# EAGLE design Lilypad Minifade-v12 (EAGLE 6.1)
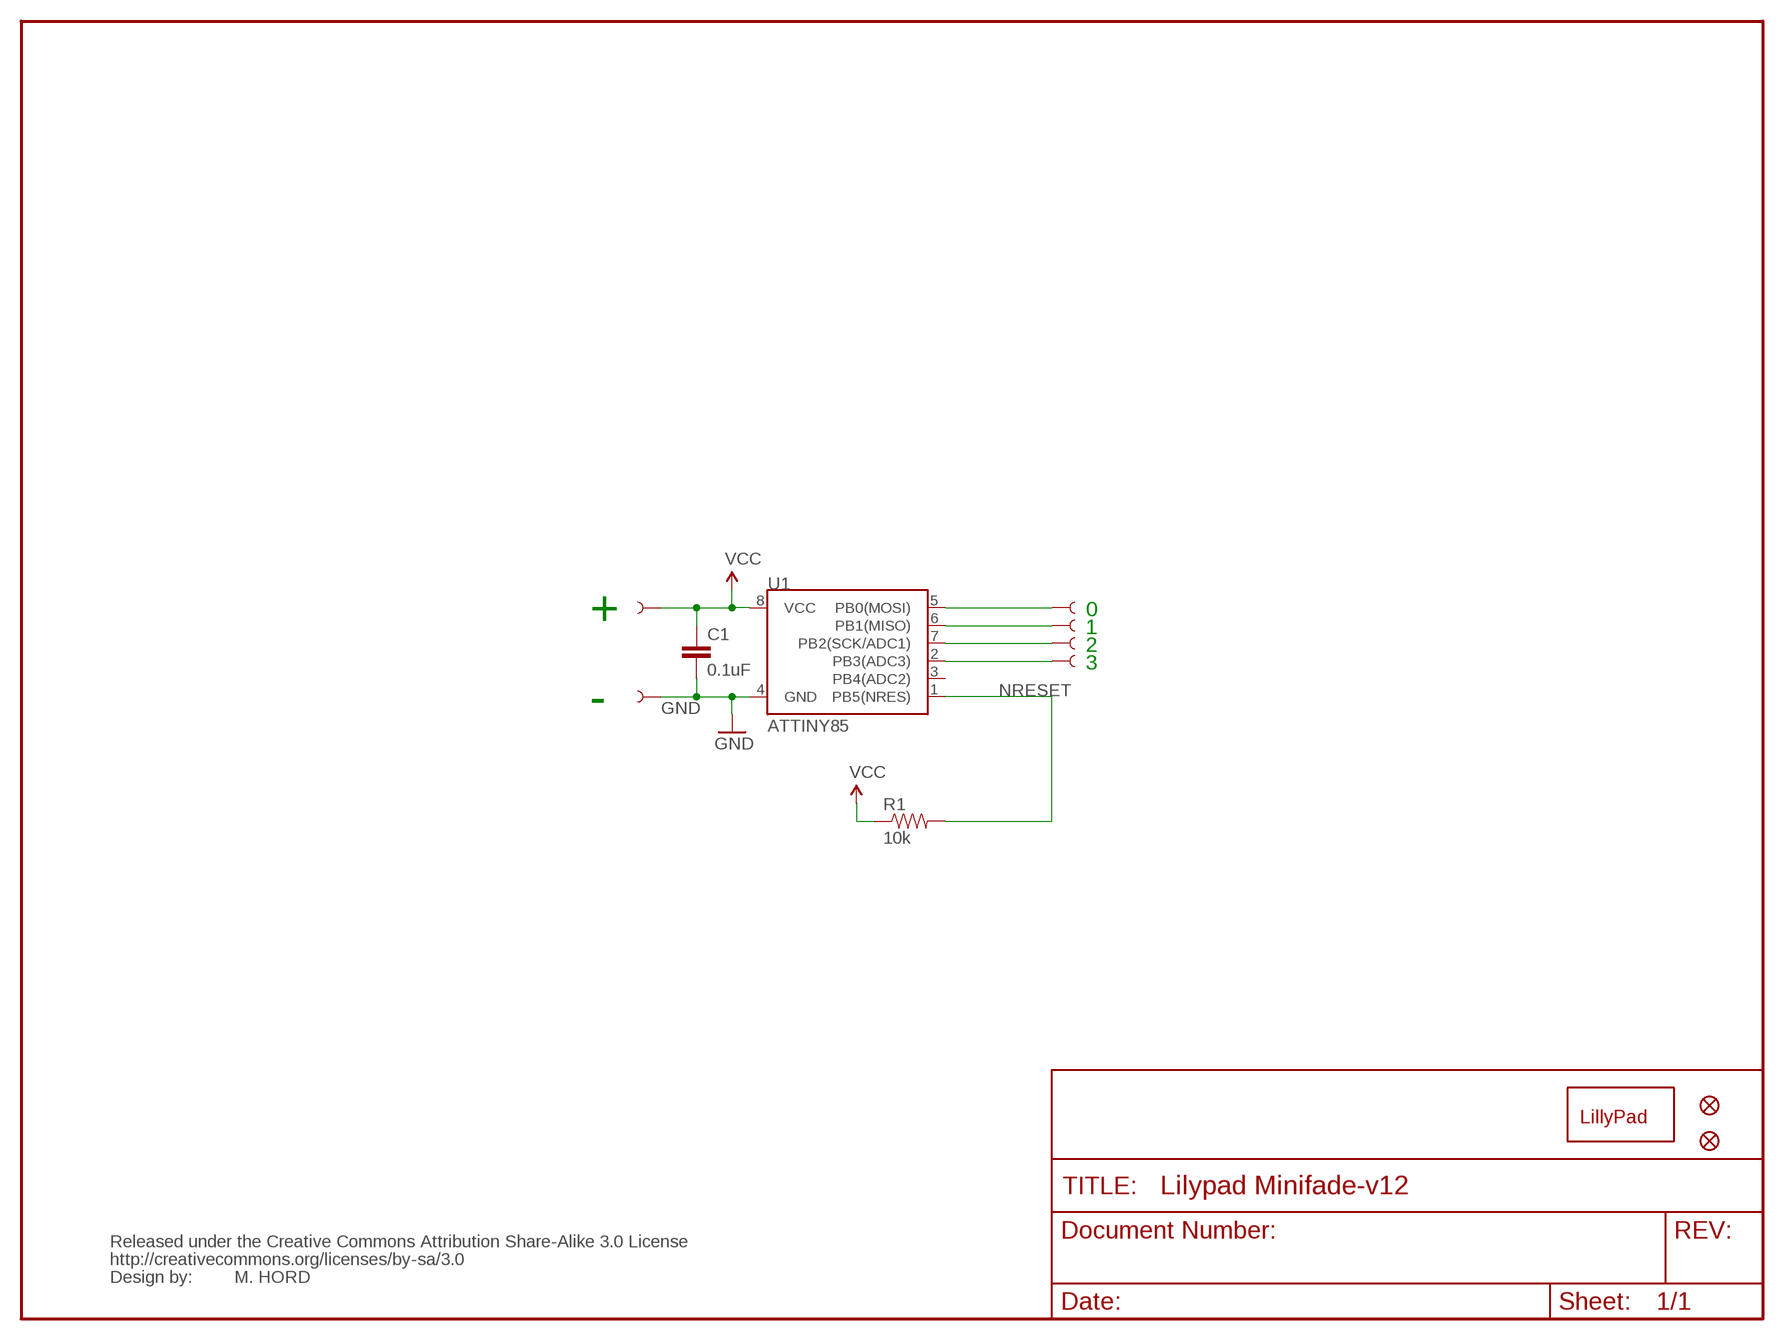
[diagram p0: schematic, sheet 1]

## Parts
C1  0.1uF  CAP0402-CAP  [0402-CAP]
JP1  FIDUCIALUFIDUCIAL  [MICRO-FIDUCIAL]
JP2  FIDUCIALUFIDUCIAL  [MICRO-FIDUCIAL]
R1  10k  RESISTOR0402-RES  [0402-RES]
U1  ATTINY85  ATTINY45  [SO08-EIAJ]
U$1  CREATIVE_COMMONS  [CREATIVE_COMMONS]
U$2  SEWTAP6  [PETAL-SMALL-2SIDE]
U$3  SEWTAP6  [PETAL-SMALL-2SIDE]
U$4  SEWTAP6  [PETAL-SMALL-2SIDE]
U$5  SEWTAP6  [PETAL-SMALL-2SIDE]
U$6  SEWTAP6  [PETAL-SMALL-2SIDE]
U$7  SEWTAP6  [PETAL-SMALL-2SIDE]
U$8  LOGO-LPL  [LOGO-L]

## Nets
GND: C1.2 U1.4(GND) U$2.1
N$3: U1.5(PB0(MOSI)) U$7.1
N$4: U1.6(PB1(MISO)) U$3.1
N$5: U1.7(PB2(SCK/ADC1)) U$4.1
N$6: U1.2(PB3(ADC3)) U$6.1
NRESET: R1.2 U1.1(PB5(NRES))
VCC: C1.1 R1.1 U1.8(VCC) U$5.1
Unconnected: U1.3(PB4(ADC2))

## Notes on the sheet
- 0
- +
- 1
- 2
- 3
- -
- M. HORD

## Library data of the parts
C1 = SparkFun:CAP: Capacitor
JP1 JP2 = SparkFun:FIDUCIAL: Fiducial Alignment Points
R1 = SparkFun:RESISTOR: Resistor
U1 = SparkFun:ATTINY45: Atmel ATTiny45
U$1 = SparkFun:CREATIVE_COMMONS
U$2-U$7 = LilyPad-Wearables:SEWTAP
U$8 = LilyPad-Wearables:LOGO-LP

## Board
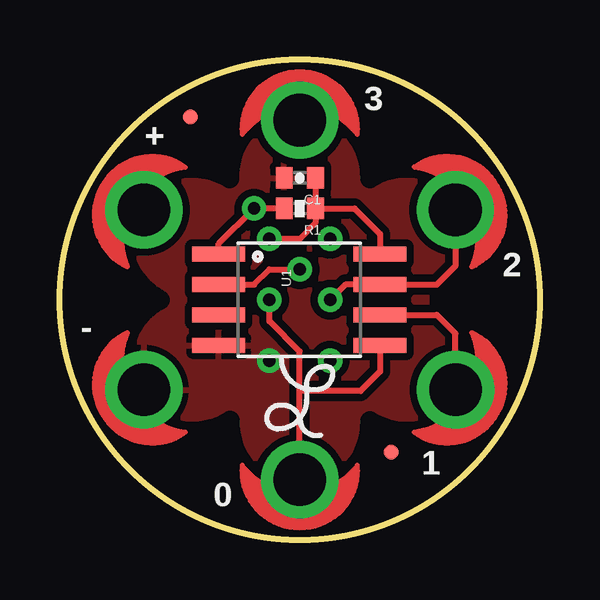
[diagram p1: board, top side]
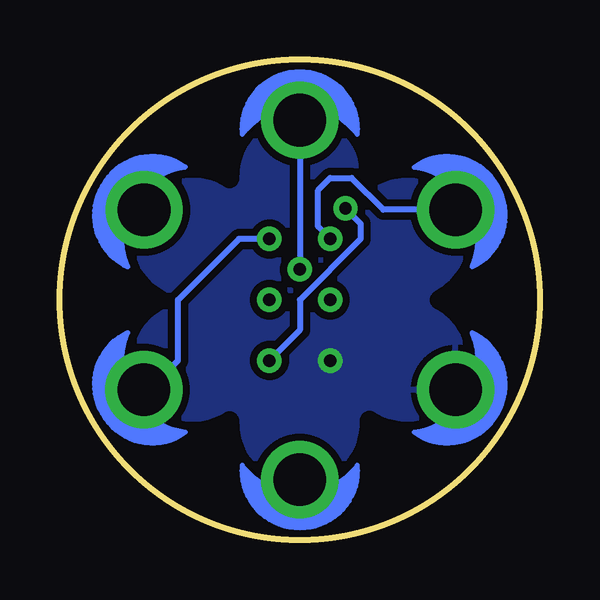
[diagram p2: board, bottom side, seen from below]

Size 20 x 20 mm. Coordinates in mm from the lower left corner, seen from the top.
Outline: circle at 10,10 radius 10
Copper layers (1*16): Top 0.035mm / dielectric 1.5mm / Bottom 0.035mm
Design rules: minimum track width 8mil, minimum drill 20mil, track to track 8mil, track to pad 8mil, pad to pad 8mil, via to via 8mil, smd to smd 8mil, copper to edge 8mil, drill to drill 8mil, minimum pad ring 12mil, minimum via ring 10mil, stop-mask expansion 4mil, vias tented up to drill 20mil, thermal gap 10mil
tRestrict: area -1,10 to 10,21; area 10,10 to 21,21; area 10,-1 to 21,10; area -1,-1 to 10,10; 6 lines
bRestrict: area -1,10 to 10,21; area 10,10 to 21,21; area 10,-1 to 21,10; area -1,-1 to 10,10; 6 lines

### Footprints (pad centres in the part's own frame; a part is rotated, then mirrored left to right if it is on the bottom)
0402-CAP = smd 0.7 x 0.9: 1 -0.65,0; 2 0.65,0
MICRO-FIDUCIAL = smd 0.635 x 0.635: 1 0,0
0402-RES = smd 0.7 x 0.9: 1 -0.65,0; 2 0.65,0
SO08-EIAJ = smd 0.61 x 2.21: 1 -1.905,-3.378; 2 -0.635,-3.378; 3 0.635,-3.378; 4 1.905,-3.378; 5 1.905,3.353; 6 0.635,3.353; 7 -0.635,3.353; 8 -1.905,3.353
PETAL-SMALL-2SIDE = drill 2.2: 1 0,0

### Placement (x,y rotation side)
C1  10,15.08 180 top
JP1  5.43,17.62 0 top
JP2  13.81,3.65 0 top
R1  10,13.81 180 top
U1  10,10 270 top
U$1  not placed on the board
U$2  3.5,6.25 300 top
U$3  16.5,6.25 60 top
U$4  16.49,13.75 120 top
U$5  3.5,13.75 240 top
U$6  10,17.49 180 top
U$7  10,2.5 0 top
U$8  10,5.94 0 top

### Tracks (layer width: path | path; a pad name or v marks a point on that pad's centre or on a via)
GND  (via drill 0.51)
  other vias: 8.73,7.46
  pour Bottom (isolate 0.305): 1.11,18.89 1.11,1.11 18.89,1.11 18.89,18.89
  pour Top (isolate 0.305): 1.11,18.89 1.11,1.11 18.89,1.11 18.89,18.89
N$3
  Top 0.254: 8.73,10 8.73,9.11 10,7.84 10,6.19 | U$7.1 10,6.19 | U1.5 13.35,7 12.54,6.19 10,6.19
N$4
  Top 0.254: U1.6 15.71,9.37 16.5,8.58 U$3.1
  Bottom 0.254: U$3.1 16.29,6.25 15.08,7.46 15.08,10
N$5
  Top 0.254: 11.27,10 11.9,10.63 U1.7 15.71,10.63 16.49,11.41 U$4.1
N$6  (via drill 0.51)
  Top 0.254: U1.2 8.1,10.63 8.73,11.27 v10,11.27
  Bottom 0.254: U$6.1 v10,11.27
N$7  (via drill 0.51)
  other vias: 8.73,10
N$8  (via drill 0.51)
  other vias: 11.27,10
N$9  (via drill 0.51)
  Bottom 0.254: v11.27,12.54 12.54,12.54 15.08,10
NRESET  (via drill 0.51)
  Top 0.254: R1.2 v8.1,13.81 6.62,12.34 U1.1
  Bottom 0.254: v8.1,13.81 7.46,13.18 7.46,12.54 10,10 10,8.73 v11.27,7.46
VCC  (via drill 0.51)
  Top 0.254: U1.8 13.35,12.74 12.29,13.81 R1.1 | C1.1 R1.1 | R1.1 10.65,13.19 10,12.54 v8.73,12.54
  Bottom 0.254: v8.73,12.54 9.24,13.05 9.24,14.57 8.73,15.08 7.84,15.08 6.51,13.75 U$5.1

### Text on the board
tPlace: 3 | + | 2 | - | 1 | 0
tValues: M. HORD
